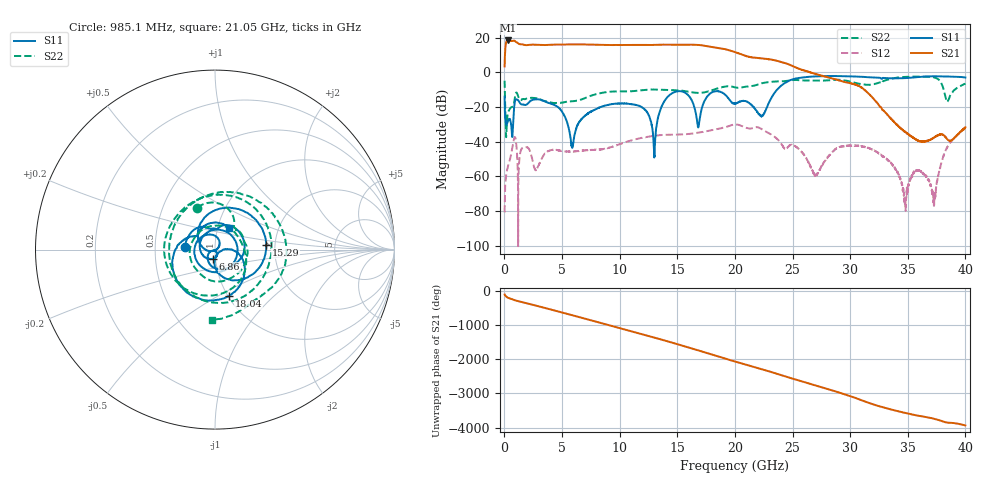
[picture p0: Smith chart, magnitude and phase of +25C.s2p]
#  HZ  S  DB  R  50.00
! Rohde & Schwarz Vector Network Analyzer
! Rohde-Schwarz,ZNB3032-4Port,1351505034101534,4.21
! Created: UTC 6/10/2026, 1:28:51 PM
! freq[Hz]  db:S11  ang:S11  db:S21  ang:S21  db:S12  ang:S12  db:S22  ang:S22
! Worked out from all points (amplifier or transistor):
!   3200 points, 10 MHz to 40 GHz, reference 50 ohm
!   highest |S21| = 18.4 dB at 285 MHz (marker M1)
!   |S21| within 3 dB of that: 93.32 MHz to 17.33 GHz (17.24 GHz wide, 198 % of centre)
!   unconditionally stable (mu >= 1): start of sweep to end of sweep
!   at 6.673 GHz: K = 13.66, MAG = 16.2 dB, |S12| = -45.1 dB
!   at 20.01 GHz: K = 3.63, MAG = 12.3 dB, |S12| = -30.0 dB
!   at 40 GHz: K = 295.13, MAG = -27.5 dB, |S12| = -32.1 dB
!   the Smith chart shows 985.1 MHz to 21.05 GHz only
!   S11 on the Smith chart (normalised r, x): 985.1 MHz: 0.71, +0.02; 6.86 GHz: 0.98, -0.10; 15.29 GHz: 1.80, +0.11; 18.04 GHz: 1.01, -0.56; 21.05 GHz: 1.14, +0.28
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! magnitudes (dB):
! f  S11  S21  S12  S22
! 10 MHz  -14.0  3.4  -80.7  -4.8
! 285 MHz  -28.3  18.4  -54.6  -23.9
! 985.1 MHz  -15.5  17.6  -39.3  -11.9
! 4.573 GHz  -19.7  16.0  -44.8  -17.6
! 5.873 GHz  -43.5  16.1  -45.7  -16.7
! 6.685 GHz  -26.8  16.1  -45.2  -15.6
! 6.86 GHz  -25.7  16.1  -45.0  -15.2
! 11.57 GHz  -19.0  15.8  -38.2  -10.6
! 13 GHz  -49.0  15.8  -36.6  -9.9
! 13.35 GHz  -25.4  15.9  -36.3  -10.0
! 15.29 GHz  -10.8  15.9  -35.8  -10.5
! 16.81 GHz  -31.7  15.8  -34.8  -11.9
! 18.04 GHz  -11.4  14.6  -33.2  -10.2
! 20.01 GHz  -18.0  11.6  -30.0  -8.7
! 21.05 GHz  -16.9  9.2  -32.1  -8.1
! 26.67 GHz  -2.4  -0.3  -56.3  -4.7
! 29.74 GHz  -2.3  -5.9  -42.3  -4.9
! 33.34 GHz  -3.4  -25.2  -50.9  -4.1
! 34.76 GHz  -3.3  -34.2  -73.0  -2.6
! 35.86 GHz  -2.7  -39.1  -56.4  -2.4
! 37.26 GHz  -2.3  -37.7  -75.2  -2.9
! 40 GHz  -3.0  -31.7  -32.1  -6.4
